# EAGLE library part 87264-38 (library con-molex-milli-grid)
RECEPTACAL
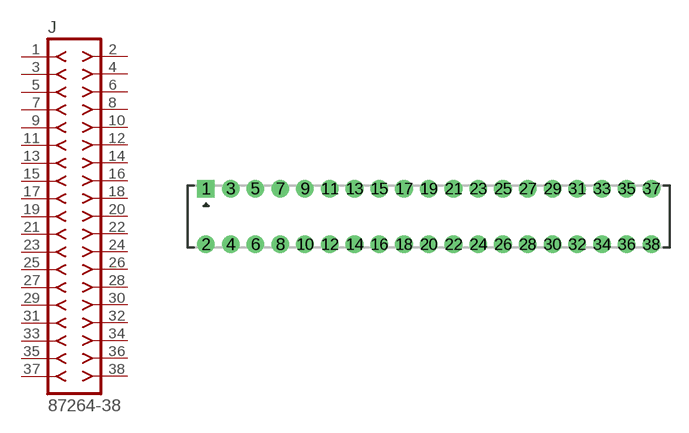
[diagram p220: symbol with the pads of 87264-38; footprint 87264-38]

Designator prefix J

## 87264-38  [87264-38]
1  1  pas
2  2  pas
3  3  pas
4  4  pas
5  5  pas
6  6  pas
7  7  pas
8  8  pas
9  9  pas
10  10  pas
11  11  pas
12  12  pas
13  13  pas
14  14  pas
15  15  pas
16  16  pas
17  17  pas
18  18  pas
19  19  pas
20  20  pas
21  21  pas
22  22  pas
23  23  pas
24  24  pas
25  25  pas
26  26  pas
27  27  pas
28  28  pas
29  29  pas
30  30  pas
31  31  pas
32  32  pas
33  33  pas
34  34  pas
35  35  pas
36  36  pas
37  37  pas
38  38  pas

## Footprint 87264-38 (pad centres in mm)
RECEPTACAL Dual Row, Side Entry
drill 0.914 square: 1 -18,2.25
drill 0.914: 2 -18,-2.25; 3 -16,2.25; 4 -16,-2.25; 5 -14,2.25; 6 -14,-2.25; 7 -12,2.25; 8 -12,-2.25; 9 -10,2.25; 10 -10,-2.25; 11 -8,2.25; 12 -8,-2.25; 13 -6,2.25; 14 -6,-2.25; 15 -4,2.25; 16 -4,-2.25; 17 -2,2.25; 18 -2,-2.25; 19 0,2.25; 20 0,-2.25; 21 2,2.25; 22 2,-2.25; 23 4,2.25; 24 4,-2.25; 25 6,2.25; 26 6,-2.25; 27 8,2.25; 28 8,-2.25; 29 10,2.25; 30 10,-2.25; 31 12,2.25; 32 12,-2.25; 33 14,2.25; 34 14,-2.25; 35 16,2.25; 36 16,-2.25; 37 18,2.25; 38 18,-2.25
